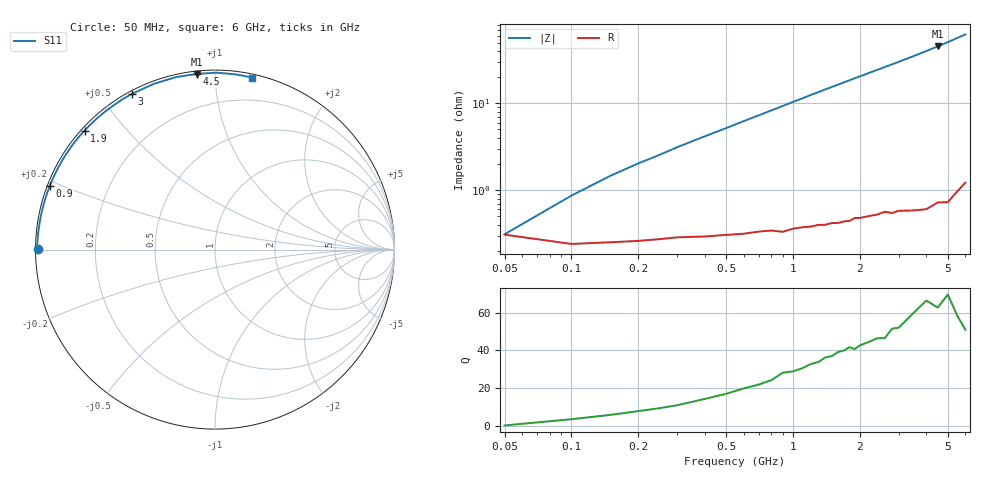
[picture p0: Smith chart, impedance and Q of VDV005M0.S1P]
! Infineon Technologies  Discrete & RF Semiconductors
! BBY 55-03
! Si Tuning Diode in SOD323
! VR =
! S-Parameters:  June  1999
# GHz  S  MA  R  50
!  f  S11
! GHz  MAG  ANG
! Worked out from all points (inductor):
!   34 points, 50 MHz to 6 GHz, reference 50 ohm
!   read as one part to ground: L = 1.53 nH near 100 MHz
!   highest Q = 66.3 at 4.5 GHz (marker M1), where L = 1.6 nH
!   S11 on the Smith chart (normalised r, x): 50 MHz: 0.01, +0.00; 900 MHz: 0.01, +0.19; 1.9 GHz: 0.01, +0.39; 3 GHz: 0.01, +0.60; 4.5 GHz: 0.01, +0.90; 6 GHz: 0.02, +1.24
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0.05  0.9878 179.9
0.1  0.9904 178.1
0.15  0.99 176.7
0.3  0.9887 172.9
0.4  0.9884 170.5
0.5  0.988 168.2
0.6  0.9877 165.8
0.8  0.9868 161.2
0.9  0.9873 158.9
1  0.9863 156.6
1.1  0.9859 154.4
1.2  0.9858 152.1
1.4  0.9854 147.8
1.6  0.985 143.7
1.7  0.9846 141.6
1.9  0.9835 137.6
2  0.9837 135.7
2.2  0.9834 131.9
2.4  0.9832 128.3
2.6  0.9825 124.7
2.8  0.9835 121.4
3  0.9831 118.0
3.5  0.9844 110.2
4  0.9854 102.7
4.5  0.9842 95.8
5  0.9857 89.4
5.5  0.9832 83.2
6  0.981 77.8
